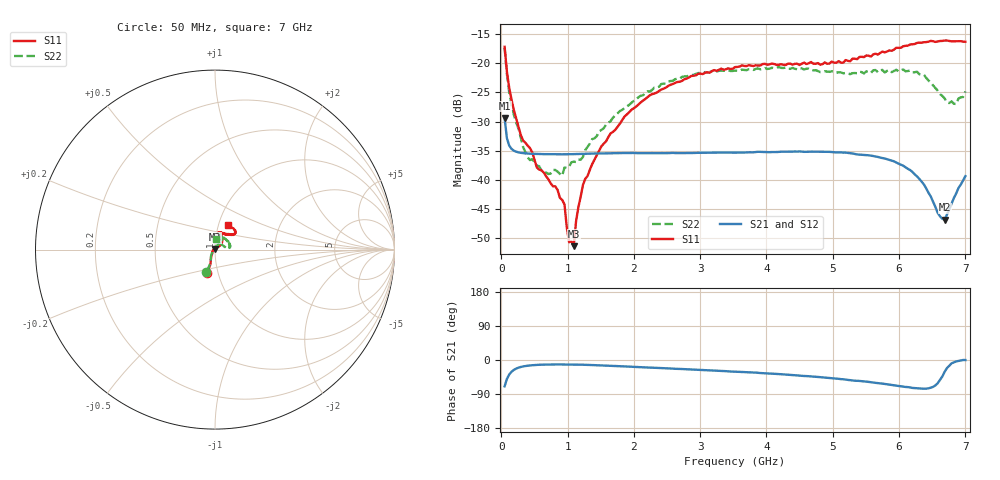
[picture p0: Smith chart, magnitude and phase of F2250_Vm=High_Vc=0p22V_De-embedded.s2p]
! Integrated Device Technology
! Corporate Headquarters
! 6024 Silver Creek Valley Road
! San Jose, CA 95138  USA
! Phone:  1-408-284-8200
! Toll Free:  1-800-223-1366
! Webpage:  http://www.idt.com/
! Timing and RF Division
! 515 Groton Road, Suite 102
! Westford, MA 01886-6024
! Device:  F2250
! Description: Voltage Variable RF Attenuator
! Frequency:  50.0 -  6000.00 MHz
! Package:  3x3 mm Thin QFN Plastic Package: 16 pin
! Ports:  2 RF, 3 DC
!  Pin  1  = GND
!  Pin  2  = NC
!  Pin  3  = RF1  = Port 1
!  Pin  4  = NC
!  Pin  5  = GND
!  Pin  6  = GND
!  Pin  7  = GND
!  Pin  8  = GND
!  Pin  9  = NC
!  Pin 10  = RF2  = Port 2
!  Pin 11  = NC
!  Pin 12  = GND
!  Pin 13  = GND
!  Pin 14  = VCNTRL
!  Pin 15  = VDD
!  Pin 16  = VMODE
! Vcntrl:  0.220 Volts
! Vmode:  +3.300 Volts
! Vdd:  +3.30  Volts
! Current:  1.243 mA
! Data:  The device was measured on a the F2250 evaluation board which has
!  individual transmission lines to the RF pins.  Data was collected
!  using a calibrated network analyzer.  The evaluation board was
!  de-embedded using a TRL calibration technique.
!  The reference plane is the edge of the package pin.
! Misc:  SN 10
!  Action Tracker AT0258
! Date Measured:  2014-11-26
! Date:  2015-10-15  MJV
! Note:
!  Integrated Device Technology supplies this data as a sample of measured
!  data at the package pin for this product.  Your particular data for this
!  product may vary.
!  Data was taken at 25 degrees C.
!  Integrated Device Technology reserves the right to change this data at anytime.
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# GHz S dB R 50
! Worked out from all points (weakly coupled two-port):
!   201 points, 50 MHz to 7 GHz, reference 50 ohm
!   highest |S21| = -29.38 dB at 50 MHz (marker M1); lowest = -46.8 dB at 6.687 GHz (marker M2)
!   lowest |S11| = -51.3 dB at 1.093 GHz (marker M3), VSWR 1.01, Z = 50 + j0.271 ohm
!   |S11| at or under -10 dB: start of sweep to end of sweep
!   |S22| runs from -39.3 to -17.4 dB; largest |S21 - S12| = 5.8e-05
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0.05  -17.18 -108.5  -29.38 -69.5  -29.38 -69.5  -17.38 -110.5
0.08475  -21.47 -107.4  -32.86 -50.1  -32.86 -50.1  -21.88 -109.0
0.15425  -26.22 -116.6  -34.68 -31.0  -34.67 -31.0  -27.11 -120.6
0.29325  -32.27 -127.5  -35.35 -18.5  -35.35 -18.5  -32.69 -133.4
0.3975  -34.11 -142.1  -35.47 -15.0  -35.48 -15.0  -36.12 -158.3
0.5365  -37.88 -154.6  -35.54 -13.0  -35.55 -12.9  -37.55 -179.9
0.64075  -38.73 -162.5  -35.57 -12.2  -35.58 -12.2  -38.94 160.4
0.91875  -43.42 155.8  -35.60 -11.8  -35.60 -11.8  -39.27 127.6
0.9535  -44.20 171.0  -35.60 -11.8  -35.60 -11.8  -37.86 124.0
1.023  -50.67 140.6  -35.58 -11.9  -35.59 -11.9  -37.71 107.7
1.0925  -51.34 88.8  -35.57 -12.0  -35.57 -12.0  -36.87 98.4
1.12725  -47.12 61.9  -35.56 -12.1  -35.56 -12.1  -36.92 91.4
1.2315  -40.87 40.9  -35.52 -12.5  -35.52 -12.5  -36.05 76.8
1.6485  -32.02 41.2  -35.43 -15.2  -35.43 -15.2  -29.92 59.8
2.37825  -24.75 46.7  -35.40 -21.1  -35.40 -21.1  -24.02 53.9
3.525  -20.66 71.7  -35.31 -30.6  -35.31 -30.6  -21.26 72.9
4.7065  -20.07 72.0  -35.16 -44.0  -35.15 -43.9  -21.22 70.3
5.85325  -17.79 40.5  -36.57 -64.9  -36.58 -64.9  -21.14 23.3
6.27025  -16.52 39.4  -39.38 -74.5  -39.39 -74.5  -21.46 8.6
6.68725  -16.11 47.9  -46.80 -31.1  -46.79 -30.9  -26.04 28.4
6.861  -16.22 54.5  -42.32 -3.8  -42.28 -3.8  -26.99 57.4
7  -16.32 62.4  -39.35 -0.1  -39.32 -0.3  -24.82 83.6
